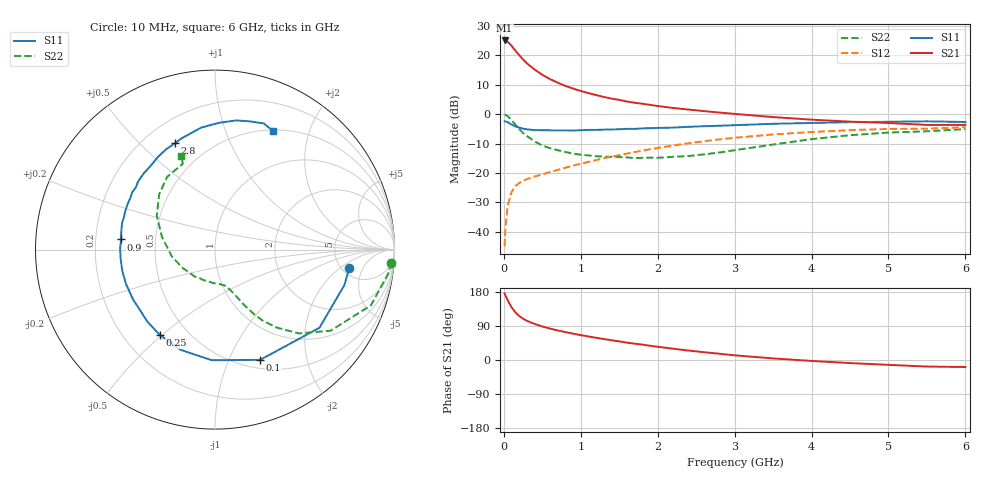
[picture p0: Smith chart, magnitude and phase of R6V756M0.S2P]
! SIEMENS Small Signal Semiconductors
! BFR193
! Si NPN RF Bipolar Junction Transistor in SOT23
! VCE = 0.75 V  IC = 6 mA
! Common Emitter S-Parameters:  May  1996
# GHz  S  MA  R  50
!  f  S11  S21  S12  S22
! GHz  MAG  ANG  MAG  ANG  MAG  ANG  MAG  ANG
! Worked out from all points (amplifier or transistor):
!   36 points, 10 MHz to 6 GHz, reference 50 ohm
!   highest |S21| = 25.0 dB at 10 MHz (marker M1)
!   |S21| within 3 dB of that: start of sweep to 136 MHz
!   unconditionally stable (mu >= 1): 817.5 MHz to 2.289 GHz
!   at 250 MHz: K = 0.49, MSG = 20.6 dB, |S12| = -22.7 dB
!   at 1.4 GHz: K = 1.07, MAG = 8.2 dB, |S12| = -14.5 dB
!   at 6 GHz: K = 0.99, MSG = 0.4 dB, |S12| = -4.5 dB
!   S11 on the Smith chart (normalised r, x): 10 MHz: 5.87, -2.73; 100 MHz: 0.60, -1.31; 250 MHz: 0.35, -0.49; 900 MHz: 0.31, +0.05; 2.8 GHz: 0.32, +0.64; 6 GHz: 0.52, +1.48
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0.01  0.7552 -7.6  17.83 175.6  0.0057 86.2  0.9839 -4.2
0.02  0.7476 -15.3  17.55 170.7  0.0113 80.5  0.9725 -8.2
0.05  0.7269 -36.8  16.94 157.5  0.0277 73.0  0.9223 -19.7
0.1  0.6639 -67.7  14.5 139.3  0.0471 60.2  0.7862 -35.1
0.15  0.6165 -91.6  11.95 125.6  0.06 52.2  0.6604 -45.0
0.2  0.5901 -109.0  10.05 116.1  0.0674 48.3  0.5546 -51.6
0.25  0.5664 -122.8  8.446 108.9  0.0733 45.8  0.4767 -56.1
0.3  0.5507 -133.0  7.279 103.4  0.0787 44.9  0.4234 -58.7
0.4  0.5343 -149.0  5.72 95.2  0.0872 45.3  0.3438 -62.5
0.5  0.5318 -159.4  4.648 88.4  0.0947 46.7  0.2926 -65.1
0.6  0.5297 -167.7  3.929 82.9  0.1037 47.9  0.2634 -67.0
0.7  0.5283 -174.4  3.419 78.0  0.1127 49.5  0.2437 -68.9
0.9  0.5266 173.8  2.714 69.5  0.133 52.0  0.2124 -73.5
1.1  0.5386 164.2  2.273 62.0  0.1542 53.4  0.1986 -79.5
1.3  0.5445 156.3  1.958 55.3  0.1775 53.6  0.1891 -85.9
1.6  0.5609 145.5  1.635 45.8  0.213 53.0  0.1834 -97.9
2.2  0.5895 127.1  1.271 29.9  0.2918 48.4  0.1882 -127.3
2.8  0.6333 110.8  1.064 16.6  0.3715 40.7  0.2223 -161.7
3.5  0.6843 96.4  0.89 4.2  0.4506 29.6  0.3038 166.6
4.5  0.7293 80.7  0.744 -8.1  0.5337 14.2  0.4377 135.3
5.5  0.7536 68.8  0.654 -17.3  0.5652 -0.7  0.5104 110.6
6  0.7345 63.7  0.657 -18.5  0.5987 -5.1  0.5563 109.7
